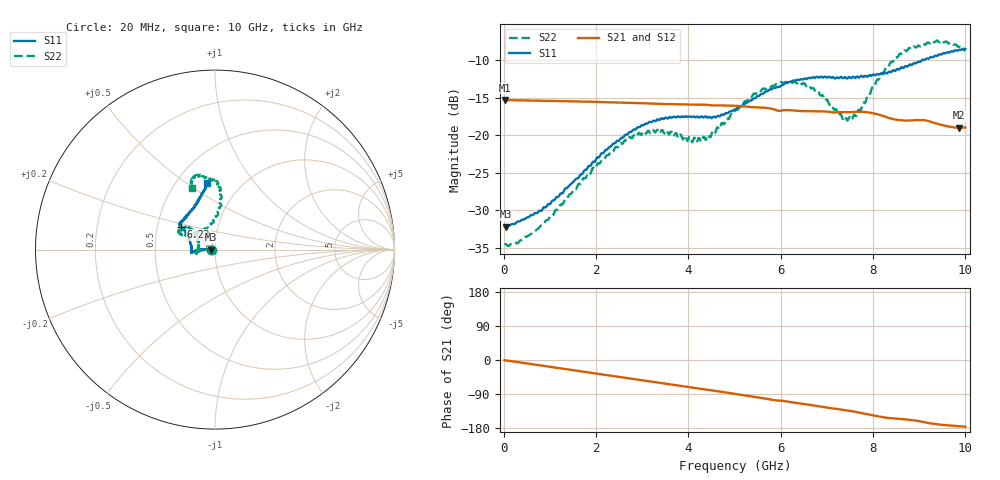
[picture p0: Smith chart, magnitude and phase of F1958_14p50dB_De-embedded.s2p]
! Integrated Device Technology
! Corporate Headquarters
! 6024 Silver Creek Valley Road
! San Jose, CA 95138  USA
! Phone:  1-408-284-8200
! Toll Free:  1-800-223-1366
! Webpage:  http://www.idt.com/
! Timing and RF Division
! 515 Groton Road, Suite 102
! Westford, MA 01886-6024
! Device:  F1958
! Description: 7-bit 0.25 dB Digital Step Attenuator
! Frequency:  0.001 -  6.000 GHz
! Package:  4x4 mm Thin QFN Plastic Package: 24 pin
! Ports:  2 RF, 12 DC
!  Pin  1  = D0
!  Pin  2  = VDD
!  Pin  3  = VMODE
!  Pin  4  = GND
!  Pin  5  = RF1  =  Port 1
!  Pin  6  = GND
!  Pin  7  = GND
!  Pin  8  = GND
!  Pin  9  = GND
!  Pin 10  = GND
!  Pin 11  = GND
!  Pin 12  = GND
!  Pin 13  = GND
!  Pin 14  = RF2  =  Port 2
!  Pin 15  = GND
!  Pin 16  = LE
!  Pin 17  = CLK
!  Pin 18  = DATA
!  Pin 19  = D6
!  Pin 20  = D5
!  Pin 21  = D4
!  Pin 22  = D3
!  Pin 23  = D2
!  Pin 24  = D1
! State:  58
! Atten State:  14.50 dB
! Voltage:  +3.30 Volts
! Current:  0.258 mA
! Data:  The device was measured on a F1958 evaluation board which has
!  individual transmission lines to the RF pins.  Data was collected
!  using a calibrated network analyzer.  The evaluation board was
!  de-embedded using Automatic Fixture Removal (AFR).
!  The reference plane is the edge of the package pin.
! Misc:
!  Action Tracker AT0419
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# GHz S dB R 50
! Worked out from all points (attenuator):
!   500 points, 20 MHz to 10 GHz, reference 50 ohm
!   highest |S21| = -15.29 dB at 20 MHz (marker M1); lowest = -19.0 dB at 9.86 GHz (marker M2)
!   lowest |S11| = -32.2 dB at 40 MHz (marker M3), VSWR 1.05, Z = 47.6 - j0.0792 ohm
!   |S11| at or under -10 dB: start of sweep to 9.056 GHz
!   |S22| runs from -34.8 to -7.4 dB; largest |S21 - S12| = 0.00064
!   S11 on the Smith chart (normalised r, x): 20 MHz: 0.95, -0.00; 6.22 GHz: 0.66, +0.18; 10 GHz: 0.70, +0.60
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0.02  -32.14 -178.1  -15.29 -0.5  -15.29 -0.5  -34.54 -177.8
0.04  -32.18 -178.1  -15.30 -0.9  -15.30 -0.8  -34.47 -176.8
0.3  -31.47 177.8  -15.34 -5.6  -15.34 -5.6  -34.39 179.6
0.72  -30.36 178.4  -15.37 -13.1  -15.37 -13.1  -32.53 -179.9
1.7  -25.15 178.7  -15.50 -30.5  -15.50 -30.5  -26.05 -179.8
2.6  -20.20 -177.9  -15.66 -46.5  -15.65 -46.5  -20.88 -175.2
2.92  -18.91 -175.3  -15.71 -52.2  -15.70 -52.3  -19.69 -171.9
3.36  -17.93 -173.1  -15.82 -60.0  -15.81 -60.1  -19.54 -167.6
4.26  -17.57 -179.5  -15.92 -75.8  -15.93 -75.9  -20.70 169.7
4.52  -17.64 174.6  -16.02 -80.6  -16.03 -80.7  -19.49 154.9
5.02  -16.57 160.9  -16.06 -89.6  -16.07 -89.6  -16.61 140.1
5.54  -14.72 150.5  -16.29 -99.3  -16.30 -99.2  -14.08 141.3
6.22  -12.86 146.5  -16.66 -111.2  -16.68 -111.2  -12.87 152.5
6.68  -12.31 144.1  -16.80 -119.2  -16.81 -119.1  -13.73 154.8
7.3  -12.22 137.7  -16.91 -130.6  -16.92 -130.5  -17.13 134.5
7.5  -12.28 134.9  -16.92 -134.4  -16.92 -134.3  -17.58 116.1
7.68  -12.24 131.9  -16.86 -138.3  -16.86 -138.3  -16.65 98.9
8.34  -11.55 116.0  -17.68 -153.0  -17.68 -153.2  -10.78 82.8
8.68  -10.90 109.3  -18.03 -156.5  -18.03 -156.5  -8.68 87.2
9.26  -9.56 101.4  -18.22 -167.5  -18.23 -167.6  -7.55 100.1
9.86  -8.62 97.0  -18.99 -174.6  -19.04 -174.5  -8.23 109.4
10  -8.51 97.0  -18.95 -176.3  -18.98 -176.2  -8.75 110.3
